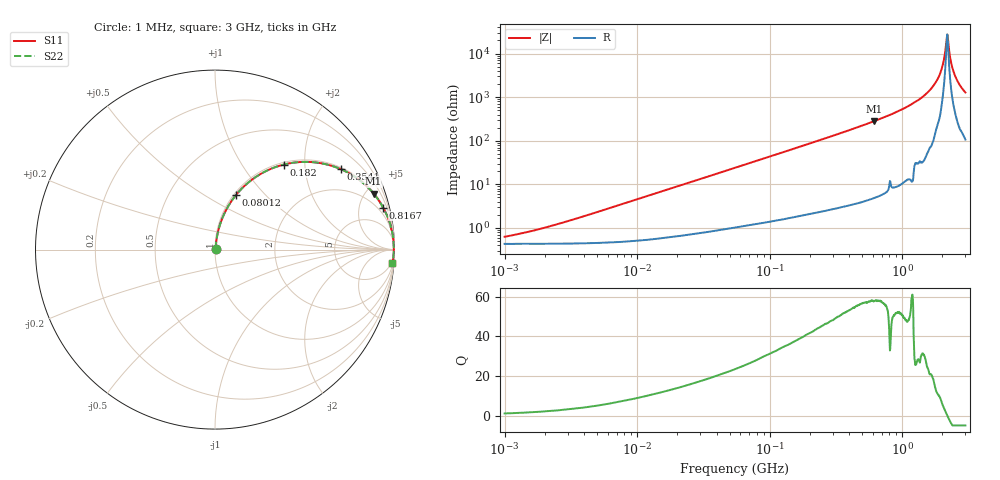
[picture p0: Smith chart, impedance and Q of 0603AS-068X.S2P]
!s-Parameter Generated by FASTRON Sdn. Bhd.
!FASTRON P/N : 0603AS-068X
!Keysight Technologies: E4991B_MY54100416_A.01.15
!Date: Wed Oct 04 11:02:20 2023
!Date created: Wed Oct 04 11:02:20 2023
!Version  : Rev01 Wed Oct 04 11:02:20 2023
!Data & Calibration Information:
!Freq	S11	S21	S12	S22
!PortZ  Port1:50+j0  Port2:50+j0
!When reading reference impedance value at option line is always used.
! Remarks : This data is being provided solely for informational purposes.
# Hz S dB R 50
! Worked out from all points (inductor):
!   1601 points, 1 MHz to 3 GHz, reference 50 ohm
!   read as one part in series: L = 72.3 nH near 2.889 MHz
!   highest Q = 58 at 614.1 MHz (marker M1), where L = 72.9 nH
!   self-resonance near 2.189 GHz
!   S11 on the Smith chart (normalised r, x): 1 MHz: 1.01, +0.01; 80.12 MHz: 1.02, +0.70; 182 MHz: 1.04, +1.57; 354.1 MHz: 1.06, +3.09; 816.7 MHz: 1.21, +7.92; 3 GHz: 3, -25
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1000000  -44.09 46.4  -0.04 -0.3  -0.04 -0.3  -44.09 46.4
3804036  -35.01 74.6  -0.04 -1.0  -0.04 -1.0  -35.01 74.6
1.447069e7  -23.81 81.3  -0.07 -3.7  -0.07 -3.7  -23.81 81.3
5.477226e7  -12.75 74.2  -0.32 -13.3  -0.32 -13.3  -12.75 74.2
8.011685e7  -9.77 69.0  -0.59 -18.9  -0.59 -18.9  -9.77 69.0
1.820241e8  -4.29 51.0  -2.19 -37.6  -2.19 -37.6  -4.29 51.0
2.083556e8  -3.60 47.3  -2.67 -41.3  -2.67 -41.3  -3.60 47.3
3.541315e8  -1.60 32.6  -5.37 -56.3  -5.37 -56.3  -1.60 32.6
6.140682e8  -0.56 19.5  -9.54 -69.5  -9.54 -69.5  -0.56 19.5
7.925923e8  -0.33 14.5  -12.04 -74.3  -12.04 -74.3  -0.33 14.5
8.167498e8  -0.32 14.1  -12.28 -74.4  -12.28 -74.4  -0.32 14.1
1.320433e9  -0.09 6.6  -18.73 -81.3  -18.73 -81.3  -0.09 6.6
1.67054e9  -0.04 3.5  -24.24 -83.7  -24.24 -83.7  -0.04 3.5
1.941122e9  -0.03 1.6  -31.16 -81.9  -31.16 -81.9  -0.03 1.6
2.03054e9  -0.03 1.0  -35.14 -77.8  -35.14 -77.8  -0.03 1.0
2.134733e9  -0.03 0.3  -43.27 -58.5  -43.27 -58.5  -0.03 0.3
2.188818e9  -0.03 0.0  -48.81 -1.6  -48.81 -1.6  -0.03 0.0
2.244273e9  -0.03 -0.3  -43.33 56.2  -43.33 56.2  -0.03 -0.3
2.359433e9  -0.04 -1.0  -34.96 75.9  -34.96 75.9  -0.04 -1.0
2.492946e9  -0.04 -1.7  -30.22 79.9  -30.22 79.9  -0.04 -1.7
2.727913e9  -0.06 -3.0  -25.49 81.3  -25.49 81.3  -0.06 -3.0
3e9  -0.08 -4.4  -22.22 80.8  -22.22 80.8  -0.08 -4.4
